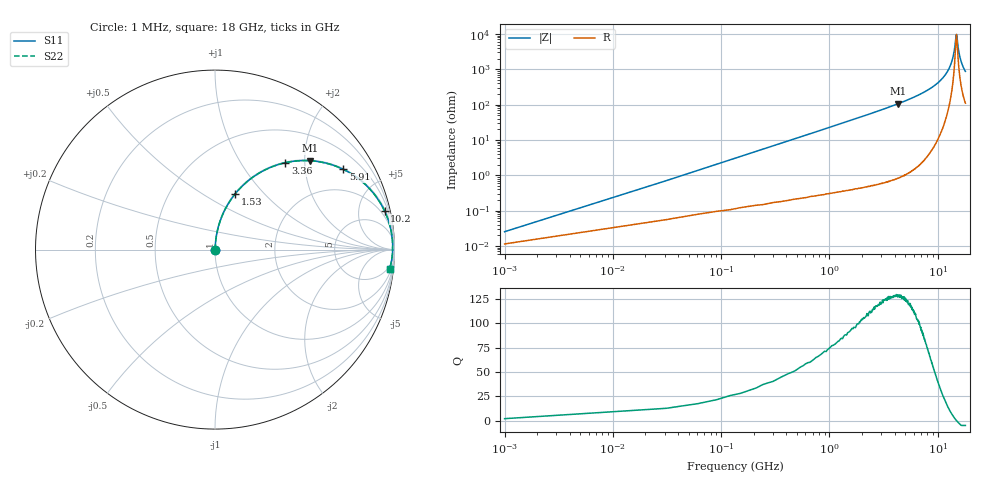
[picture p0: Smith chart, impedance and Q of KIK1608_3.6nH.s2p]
!version-2
!date-01.2022
!Series
# MHz S RI R 50
!Freq ReS11 ImS11 ReS21 ImS21 ReS12 ImS12 ReS22 ImS22
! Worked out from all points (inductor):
!   601 points, 1 MHz to 18 GHz, reference 50 ohm
!   read as one part in series: L = 3.6 nH near 91 MHz
!   highest Q = 129 at 4.29 GHz (marker M1), where L = 3.93 nH
!   self-resonance near 14.88 GHz
!   S11 on the Smith chart (normalised r, x): 1 MHz: 1.00, +0.00; 1.53 GHz: 1.01, +0.70; 3.36 GHz: 1.01, +1.60; 5.91 GHz: 1.03, +3.17; 10.2 GHz: 1.23, +8.69; 18 GHz: 3, -17
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1  0.000129 0.000226  0.9999 -0.000226  0.9999 -0.000226  0.000129 0.000226
121  0.00182 0.0273  0.9982 -0.0273  0.9982 -0.0273  0.00182 0.0273
181  0.00297 0.0408  0.997 -0.0408  0.997 -0.0408  0.00297 0.0408
301  0.00627 0.0676  0.9937 -0.0676  0.9937 -0.0676  0.00627 0.0676
481  0.0138 0.1072  0.9862 -0.1072  0.9862 -0.1072  0.0138 0.1072
751  0.0306 0.1647  0.9694 -0.1647  0.9694 -0.1647  0.0306 0.1647
1530  0.1118 0.3097  0.8882 -0.3097  0.8882 -0.3097  0.1118 0.3097
3030  0.3397 0.4695  0.6603 -0.4695  0.6603 -0.4695  0.3397 0.4695
3360  0.3917 0.4841  0.6083 -0.4841  0.6083 -0.4841  0.3917 0.4841
4290  0.5282 0.4953  0.4718 -0.4953  0.4718 -0.4953  0.5282 0.4953
5910  0.7142 0.4474  0.2858 -0.4474  0.2858 -0.4474  0.7142 0.4474
6030  0.7252 0.442  0.2748 -0.442  0.2748 -0.442  0.7252 0.442
9030  0.9084 0.2795  0.0916 -0.2795  0.0916 -0.2795  0.9084 0.2795
10200  0.9445 0.2159  0.0555 -0.2159  0.0555 -0.2159  0.9445 0.2159
12030  0.9769 0.1238  0.0231 -0.1238  0.0231 -0.1238  0.9769 0.1238
13620  0.9884 0.052  0.0116 -0.052  0.0116 -0.052  0.9884 0.052
14220  0.9898 0.0269  0.0102 -0.0269  0.0102 -0.0269  0.9898 0.0269
14790  0.9899 0.00404  0.0101 -0.00404  0.0101 -0.00404  0.9899 0.00404
15030  0.9896 -0.00531  0.0104 0.00531  0.0104 0.00531  0.9896 -0.00531
15540  0.9884 -0.0246  0.0115 0.0246  0.0115 0.0246  0.9884 -0.0246
16110  0.9863 -0.0454  0.0137 0.0454  0.0137 0.0454  0.9863 -0.0454
18000  0.9738 -0.1084  0.0262 0.1084  0.0262 0.1084  0.9738 -0.1084
